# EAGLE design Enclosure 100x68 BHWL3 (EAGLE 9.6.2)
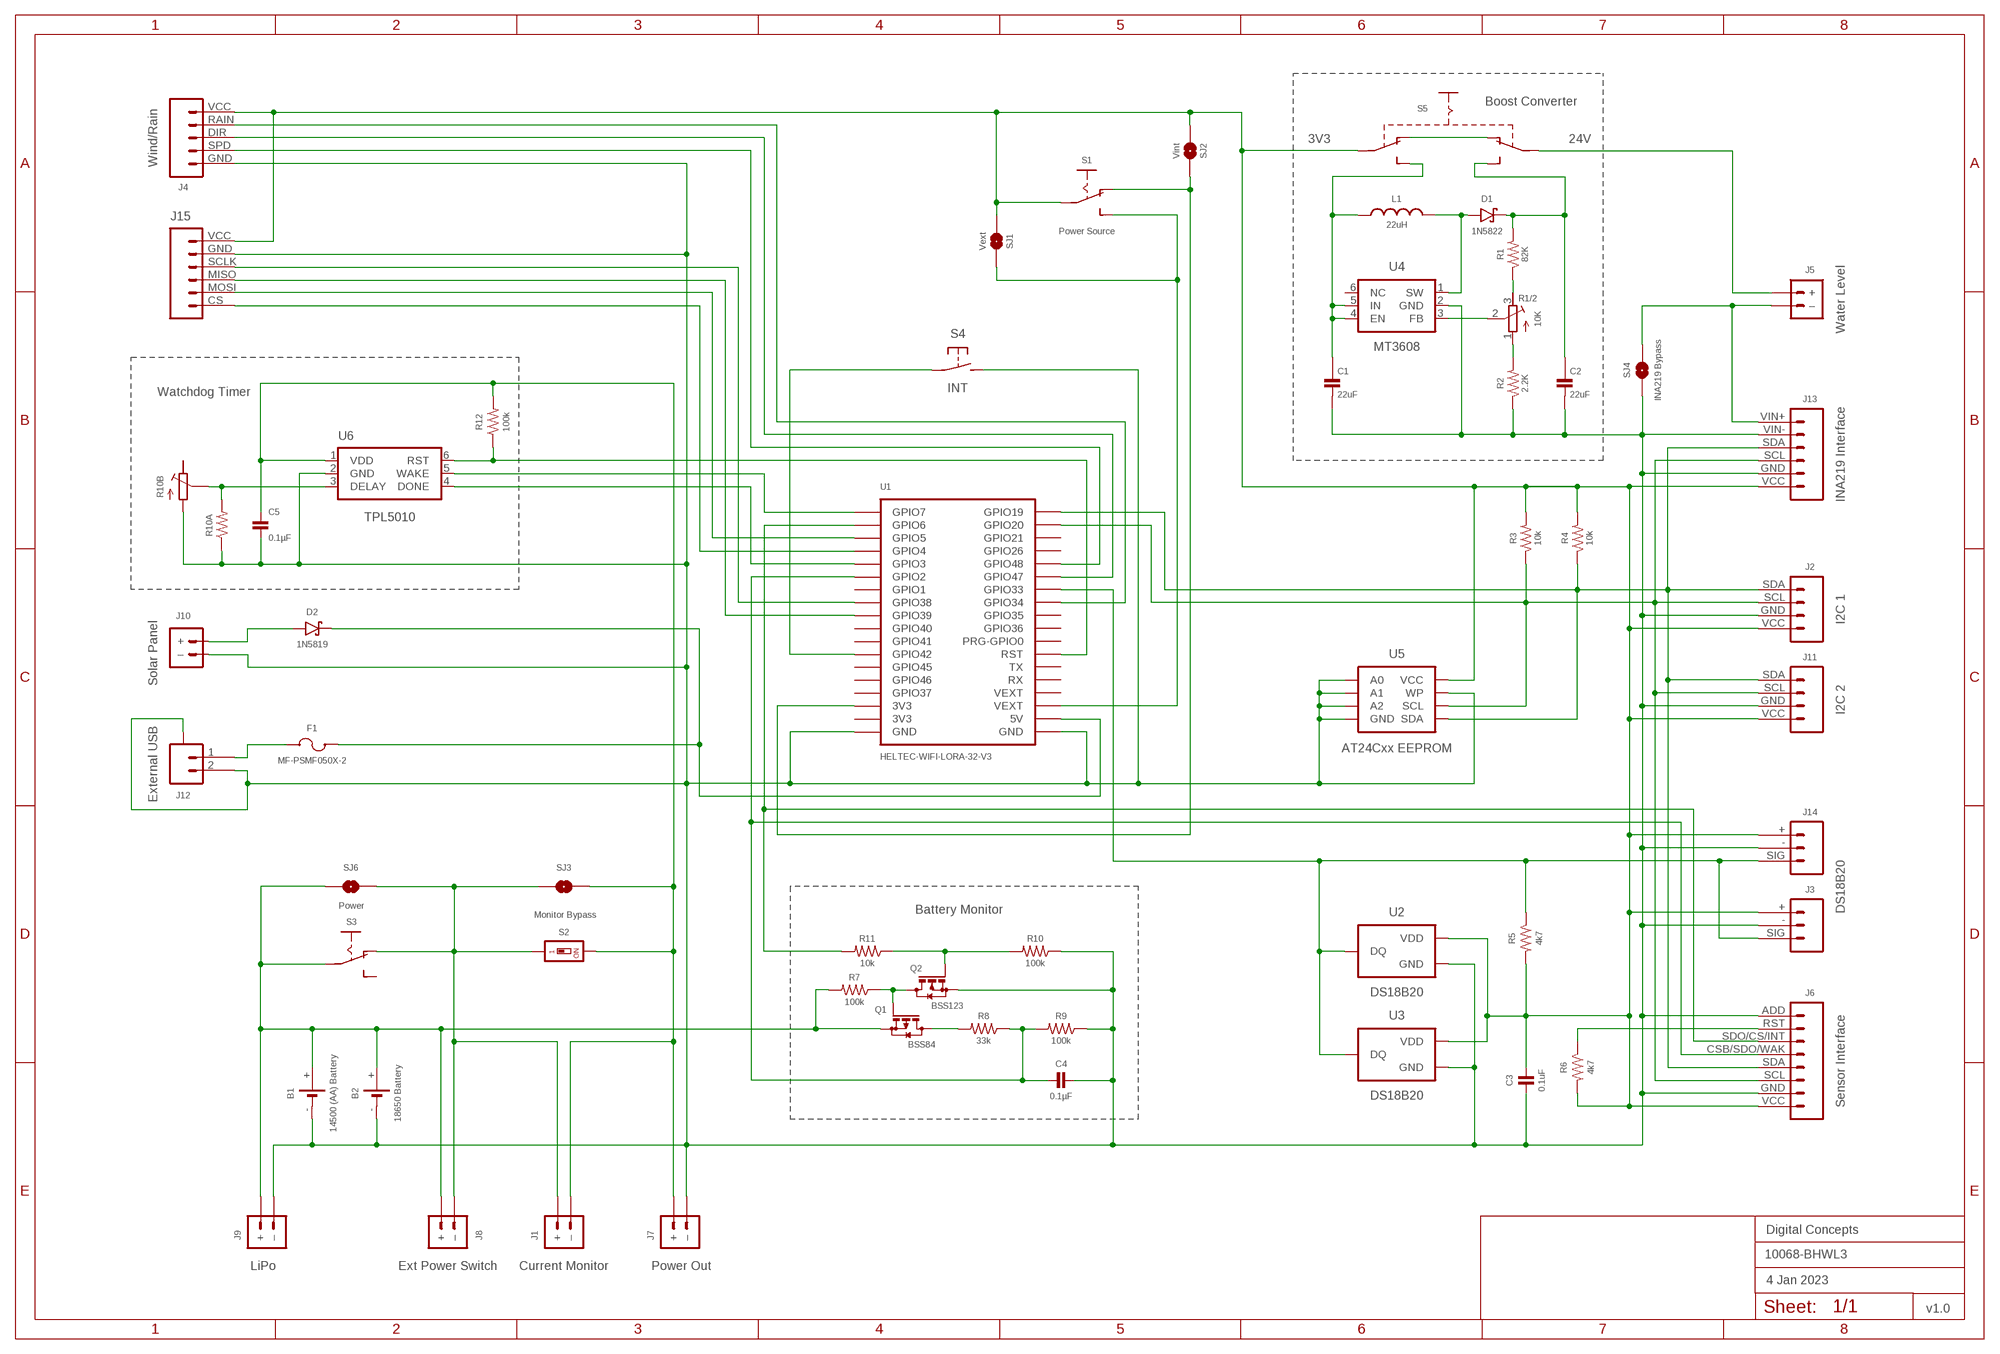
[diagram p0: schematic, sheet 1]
FRAME2 (A3L-LOC): DATE: 4 Jan 2023; OWNER: Digital Concepts; TITLE: 10068-BHWL3; VERSION: v1.0

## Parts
B1  14500 (AA) Battery  BATTERY-HOLDER-14500(AA)  [BATTERY-14500]
B2  18650 Battery  BATTERY-HOLDER-18650  [BATTERY-18650]
C1  22uF  CAPACITOR-1206  [C1206]
C2  22uF  CAPACITOR-1206  [C1206]
C3  0.1uF  CAPACITOR-0805  [C0805]
C4  0.1µF  CAPACITOR-0805  [C0805]
C5  0.1µF  CAPACITOR-0805  [C0805]
D1  1N5822  DIODE-SCHOTTKY-1N5822  [DIODE_SMB]
D2  1N5819  1N5819-SOD-123  [SOD-123]
F1  MF-PSMF050X-2  [F0805]
J1  Current Monitor  JST-PH2.0-2-HORIZONTALJST-PTH-2  [JST-PH2.0-2-HORIZONTAL]
J2  I2C 1  JST-PH2.0-4-VERTICAL-I2C  [JST-PH2.0-4-VERTICAL-I2C]
J3  DS18B20  JST-PH2.0-3-VERTICAL-DS18B20  [JST-PH2.0-3-VERTICAL-SIG]
J4  Wind/Rain  JST-PH2.0-5-DUAL-WEATHER  [JST-PH2.0-5-DUAL-WEATHER]
J5  Water Level  JST-PH2.0-2-DUAL-POWERJST-PTH-2  [JST-PH2.0-2-DUAL-POWER]
J6  Sensor Interface  HEADER-1X8-SENSOR  [CONN_08-SENSOR]
J7  Power Out  JST-GH1.25-2-HORIZONTAL-POWER  [JST-GH1.25-2-HORIZONTAL]
J8  Ext Power Switch  JST-PH2.0-2-DUAL-POWERJST-PTH-2  [JST-PH2.0-2-DUAL-POWER]
J9  LiPo  JST-PH2.0-2-HORIZONTAL-POWERJST-PTH-2  [JST-PH2.0-2-HORIZONTAL-POWER]
J10  Solar Panel  JST-PH2.0-2-VERTICAL  [JST-PH2.0-2-VERTICAL=POWER]
J11  I2C 2  JST-PH2.0-I2C-MALE-HORIZONTAL  [JST-PH2.0-4-HORIZONTAL]
J12  External USB  JST-SH1.0-2-SMD-HORIZONTAL  [JST-SH1.0-2-HORIZONTAL]
J13  INA219 Interface  INA219-I2C-MODULE  [CONN_06-INA219]
J14  JST-PH2.0-3-HORIZONTAL-DS18B20  [JST-PH2.0-DS18B20-HORIZONTAL]
J15  JST-PH2.0-6-HORIZONTAL-SPI  [JST-PH2.0-6-HORIZONTAL-SPI]
L1  22uH  INDUCTOR-CDRH104R/6D28L5038P  [CDRH104R+6D28]
Q1  BSS84  [SOT23-3]
Q2  BSS123  MOSFET-BSS123  [SOT23-3]
R1  82K  RESISTORR0805  [R0805]
R1/2  10K  RESISTOR-TRIMM-BAOTER-HORIZONTAL  [RTRIM64P]
R2  2.2K  RESISTORR0805  [R0805]
R3  10k  RESISTORR0805  [R0805]
R4  10k  RESISTORR0805  [R0805]
R5  4k7  RESISTORR0805  [R0805]
R6  4k7  RESISTORR0805  [R0805]
R7  100k  RESISTORR0805  [R0805]
R8  33k  RESISTORR0805  [R0805]
R9  100k  RESISTORR0805  [R0805]
R10  100k  RESISTORR0805  [R0805]
R10A  RESISTORR0805  [R0805]
R10B  RESISTOR-TRIMM-33  [RTRIM3*3]
R11  10k  RESISTORR0805  [R0805]
R12  100k  RESISTORR0805  [R0805]
S1  Power Source  SWITCH-SLIDE-SPDT-SMT  [SWITCH-SPDT-SMT]
S2  Monitor Bypass  SWITCH-DIP-SWS001  [SMD-001]
S3  Power  SWITCH-SLIDE-SPDT-PTH  [SWITCH-SPDT-PTH]
S4  INT  SWITCH-MOMENTARY-2-PIN  [SWITCH-2-PAD]
S5  SWITCH-SLIDE-DPDT-PTH-S  [SWITCH-DPDT-PTH]
SJ1  Vext  SJ  [SJ]
SJ2  Vint  SJ-V-2  [SJ-VIA-2]
SJ3  Monitor  SJ  [SJ]
SJ4  INA219 Bypass  SJ  [SJ]
SJ6  Power  SJ  [SJ]
U1  HELTEC-WIFI-LORA-32-V3  [HELTEC-WIFI-LORA-32-V3]
U2  DS18B20  THERMOMETER-DS18B20  [TO-92]
U3  DS18B20  THERMOMETER-DS18B20  [TO-92]
U4  MT3608  [SOT-23-6@1]
U5  AT24Cxx EEPROM  AT24CXX-EEPROM  [SOP-8]
U6  TPL5010  TPL5010DDCR  [SOT-23-6]

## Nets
GND: B1.- B2.- C1.2 C2.2 C3.2 C4.2 C5.2 J2.GND J3.- J4.GND J6.ADD J6.GND J7.-(–) J9.-(–) J10.-(–) J11.GND J12.2 J12.A@1(A) J12.A@2(A) J13.GND J13.VIN- J14.- J15.GND Q2.2(S) R2.1 R9.1 R10.1 R10A.1 R10B.1(A) S4.P$2(S) SJ4.1 U1.GND@1(GND) U1.GND@36(GND) U2.1(GND) U3.1(GND) U4.2(GND) U5.P$1(A0) U5.P$2(A1) U5.P$3(A2) U5.P$4(GND) U5.P$7(WP) U6.2(GND)
N$1: D2.A J10.+
N$2: J3.SIG J14.SIG R5.1 U1.GPIO33 U2.2(DQ) U3.2(DQ)
N$3: C4.1 J6.CSB/SDO/WAK R8.1 R9.2 U1.GPIO2
N$4: J2.SCL J6.SCL J11.SCL J13.SCL R3.1 U1.GPIO20 U5.P$6(SCL)
N$5: D2.C F1.1 U1.5V
N$6: D1.A L1.1 U4.1(SW)
N$7: Q1.3(D) R8.2
N$9: J6.RST R6.1
N$10: C5.1 J1.2(–) J7.+ R12.2 S2.2 SJ3.1 U6.1(VDD)
N$11: J2.SDA J6.SDA J11.SDA J13.SDA R4.1 U1.GPIO19 U5.P$5(SDA)
N$12: U1.GPIO7 U6.5(WAKE)
N$13: S1.3(S) SJ1.1 U1.VEXT@3(VEXT)
N$14: F1.2 J12.1
N$15: J5.-(–) J13.VIN+ SJ4.2
N$16: S4.P$1(P) U1.GPIO42
N$17: R1.1 R1/2.3(E)
N$18: R10A.2 R10B.2(S) U6.3(DELAY)
N$19: S1.1(O) SJ2.1 U1.3V3@34(3V3)
N$20: J5.+ S5.P$2(P1)
N$21: J1.1(+) J8.-(–) S2.1 S3.1(O) SJ3.2 SJ6.1
N$22: R1/2.2(S) U4.3(FB)
N$23: R1/2.1(A) R2.2
N$24: U1.GPIO3 U6.4(DONE)
N$25: C1.1 L1.2 S5.P$6(S2) U4.4(EN) U4.5(IN)
N$26: S5.P$1(O1) S5.P$4(O2)
N$27: J15.SCLK U1.GPIO38
N$28: C2.1 D1.C R1.2 S5.P$3(S1)
N$29: J15.MOSI U1.GPIO5
N$30: B1.+ B2.+ J8.+ J9.+ Q1.2(S) R7.2 S3.2(P) SJ6.2
N$31: J15.MISO U1.GPIO39
N$32: J6.SDO/CS/INT R11.2 U1.GPIO6
N$33: J15.CS U1.GPIO4
N$34: R12.1 U1.RST U6.6(RST)
N$35: Q1.1(G) Q2.3(D) R7.1
N$37: Q2.1(G) R10.2 R11.1
N$38: J4.SPD U1.GPIO48
N$39: J4.DIR U1.GPIO47
N$40: J4.RAIN U1.GPIO34
VEXT: C3.1 J2.VCC J3.+ J4.VCC J6.VCC J11.VCC J13.VCC J14.+ J15.VCC R3.2 R4.2 R5.2 R6.2 S1.2(P) S5.P$5(P2) SJ1.2 SJ2.2 SJ2.2@V U2.3(VDD) U3.3(VDD) U5.P$8(VCC)
Unconnected: R10B.3(E) S3.3(S) U1.3V3@35(3V3) U1.GPIO0(PRG-GPIO0) U1.GPIO1 U1.GPIO21 U1.GPIO26 U1.GPIO35 U1.GPIO36 U1.GPIO37 U1.GPIO40 U1.GPIO41 U1.GPIO45 U1.GPIO46 U1.RX U1.TX U1.VEXT@4(VEXT) U4.6(NC)

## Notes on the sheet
- Boost Converter
- 3V3 | 24V
- Watchdog Timer
- Battery Monitor

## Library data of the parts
B1 = digitalconcepts:BATTERY-HOLDER-14500(AA): 14500 (AA) battery holder
B2 = digitalconcepts:BATTERY-HOLDER-18650: 18650 Battery Holder
C1 C2 = digitalconcepts:CAPACITOR-1206: 1206 Capacitor
C3-C5 = digitalconcepts:CAPACITOR-0805: 0805 Capacitor
D1 = digitalconcepts:DIODE-SCHOTTKY-1N5822: 1N5822 Schottky Diode SMB
D2 = digitalconcepts:1N5819-SOD-123: 1N5819 Schottky Diode SOD-123
F1 = digitalconcepts:MF-PSMF050X-2: PTC Resettable Fuse
J1 = digitalconcepts:JST-PH2.0-2-HORIZONTAL: PH2.0 2P Right Angle PCB Connector; PROD_ID: CONN-09863; SKU: PRT-09914
J2 = digitalconcepts:JST-PH2.0-4-VERTICAL-I2C: PH2.0 4P I2C Vertical Connector
J3 = digitalconcepts:JST-PH2.0-3-VERTICAL-DS18B20: DS18B20 PH2.0 Vertical PCB Connector
J4 = digitalconcepts:JST-PH2.0-5-DUAL-WEATHER: PH2.0 5P Dual Connector
J5 J8 = digitalconcepts:JST-PH2.0-2-DUAL-POWER: JST PH2.0 2P PTH Dual-Side Connector (Power); PROD_ID: CONN-09863; SKU: PRT-09914
J6 = digitalconcepts:HEADER-1X8-SENSOR: IoT Sensors 1x8 Pin Header for 'Sandwich' IoT Sensors
J7 = digitalconcepts:JST-GH1.25-2-HORIZONTAL-POWER: JST GH1.25 2P PTH Connector (Power)
J9 = digitalconcepts:JST-PH2.0-2-HORIZONTAL-POWER: PH2.0 2P Right Angle PCB Connector; PROD_ID: CONN-09863; SKU: PRT-09914
J10 = digitalconcepts:JST-PH2.0-2-VERTICAL: PH2.0 2P PCB Connector
J11 = digitalconcepts:JST-PH2.0-I2C-MALE-HORIZONTAL: PH2.0 4P (I2C) Right Angle PCB Connector
J12 = digitalconcepts:JST-SH1.0-2-SMD-HORIZONTAL: JST SH1.0 2P SMD Horizontal Connector
J13 = digitalconcepts:INA219-I2C-MODULE: INA219 I2C Module
J14 = digitalconcepts:JST-PH2.0-3-HORIZONTAL-DS18B20: DS18B20 PH2.0 Right Angle PCB Connector
J15 = digitalconcepts:JST-PH2.0-6-HORIZONTAL-SPI: PH2.0 6P Horizontal Connector—SPI
L1 = digitalconcepts:INDUCTOR-CDRH104R/6D28: Inductor; SPICEPREFIX: L
Q1 = digitalconcepts:BSS84: P-CHANNEL MOS FET
Q2 = digitalconcepts:MOSFET-BSS123: N-CHANNEL MOS FET
R1-R10 R10A R11 R12 = digitalconcepts:RESISTOR: Resistor; SPICEPREFIX: R
R1/2 = digitalconcepts:RESISTOR-TRIMM-BAOTER-HORIZONTAL: Trimm Resistor - Horizontal BAOTER
R10B = digitalconcepts:RESISTOR-TRIMM-3*3: Trimm Resistor - 3*3 SMD
S1 = digitalconcepts:SWITCH-SLIDE-SPDT-SMT: Mini Sliding Switch SPDT SMT
S2 = digitalconcepts:SWITCH-DIP-SWS001: SMD Dip Switch 1 pol.
S3 = digitalconcepts:SWITCH-SLIDE-SPDT-PTH: Mini Sliding Switch SPDT PTH
S4 = digitalconcepts:SWITCH-MOMENTARY-2-PIN: 2 Pin Momentary Switch
S5 = digitalconcepts:SWITCH-SLIDE-DPDT-PTH-S: Switch DPDT PTH-S
SJ1 SJ3 SJ4 SJ6 = digitalconcepts:SJ: Solder Jumper
SJ2 = digitalconcepts:SJ-V-2: Solder Jumper with Pad Vias
U1 = digitalconcepts:HELTEC-WIFI-LORA-32-V3: Heltec WiFi LoRa 32 Development Board V3
U2 U3 = digitalconcepts:THERMOMETER-DS18B20: Digital Thermometer -55C-125C TO92-3; AVAILABILITY: Bad; DESCRIPTION: Temperature Sensor Digital, Local -55°C ~ 125°C 12 b 8-uMAX; MF: Maxim Integrated; MP: DS18B20; PACKAGE: TO-92 Maxim Integrated; PRICE: None
U4 = digitalconcepts:MT3608: MT3608 DC-DC Step-Up Voltage Converter
U5 = digitalconcepts:AT24CXX-EEPROM: AT24Cxx EEPROM SOP-8
U6 = digitalconcepts:TPL5010DDCR: TPL5010 Nano-Power System Timer with Watchdog

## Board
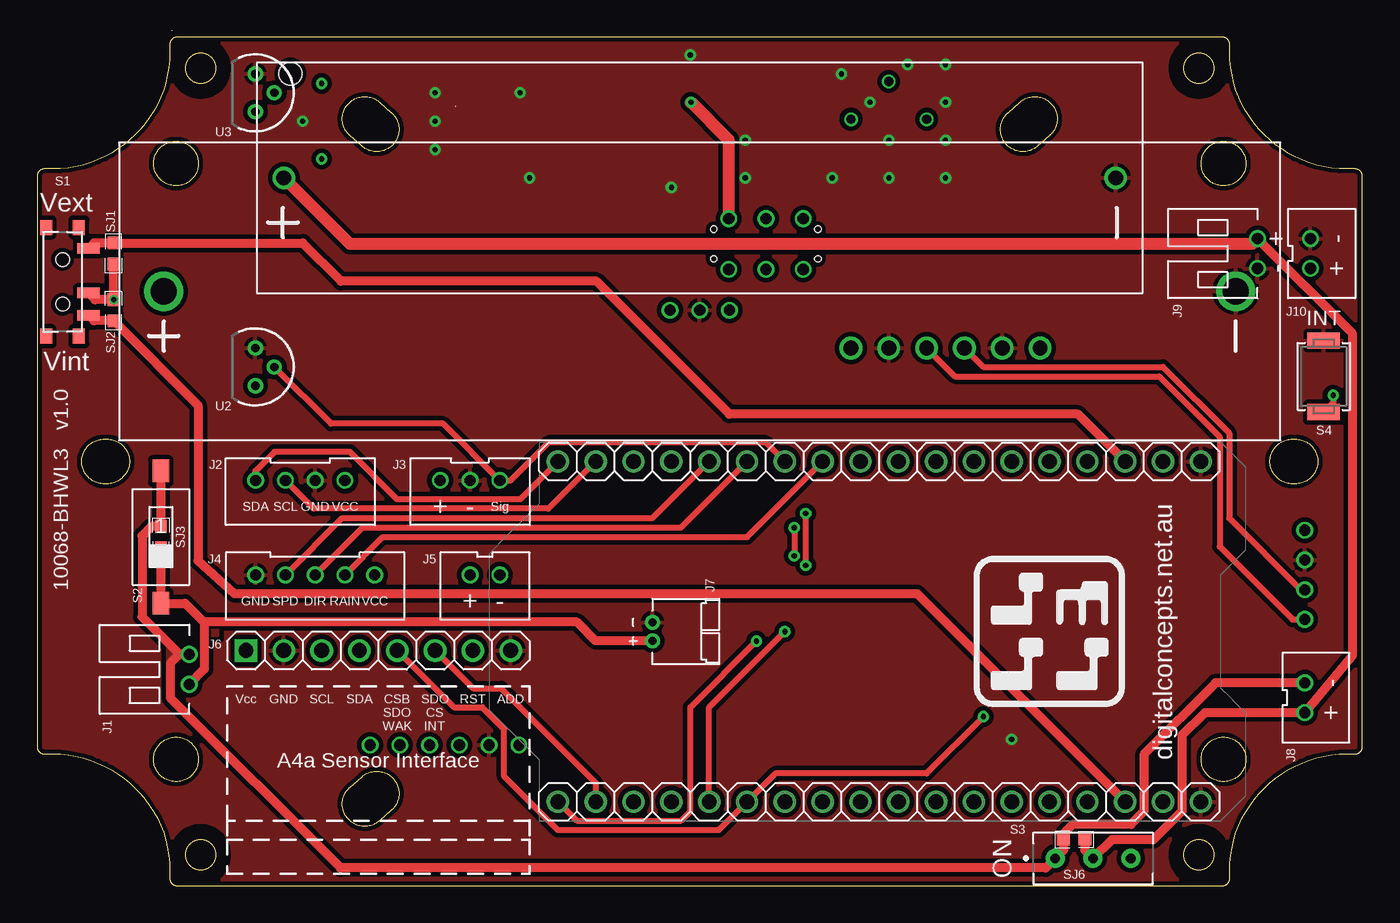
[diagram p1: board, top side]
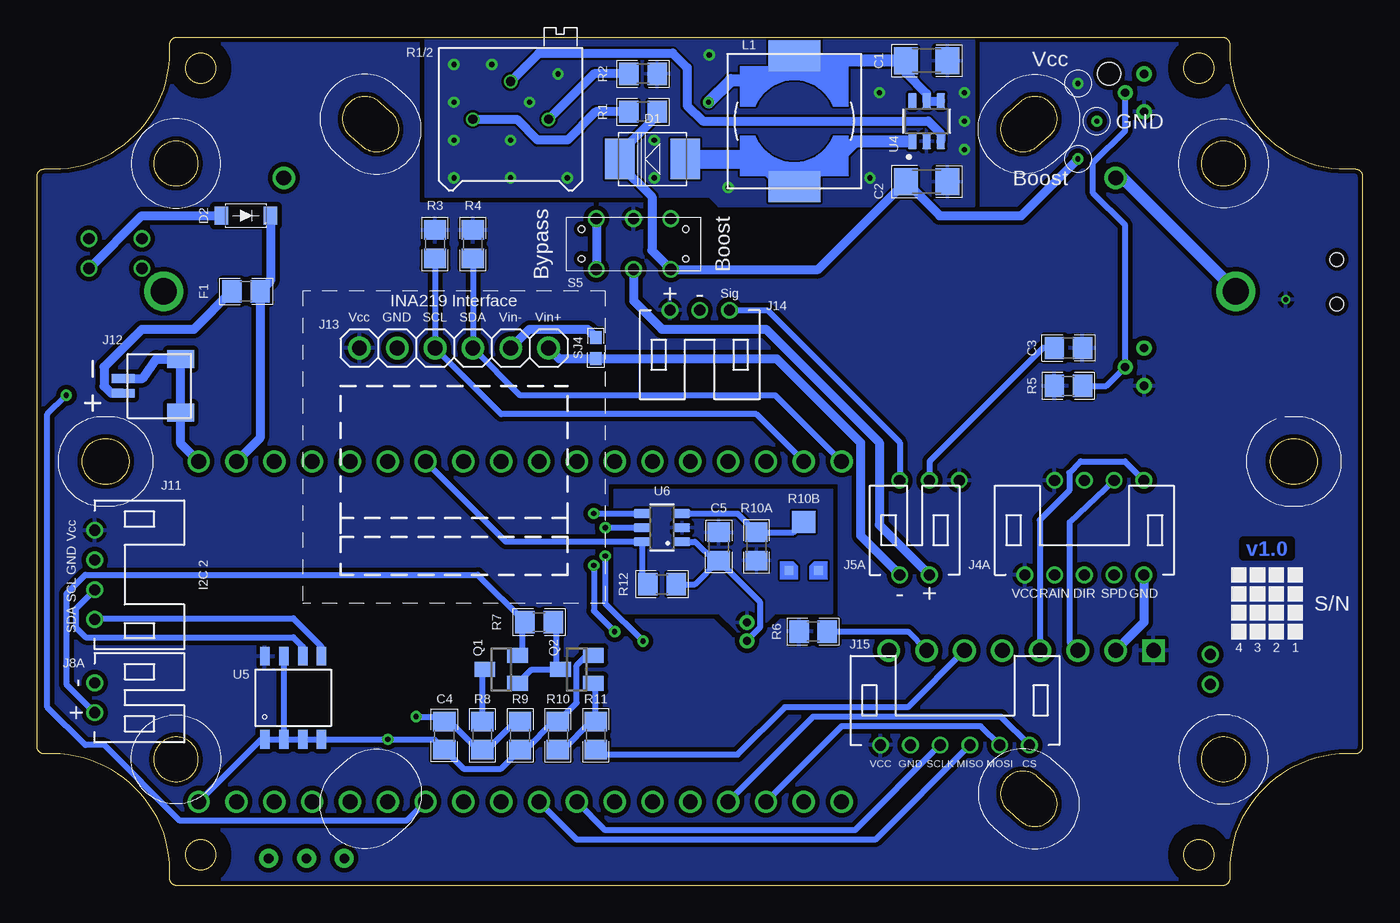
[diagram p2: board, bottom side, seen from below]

Size 89 x 57 mm. Coordinates in mm from the lower left corner, seen from the top.
Outline: 1134 segments
Outline: circle at 10.97,2.08 radius 1.02
Outline: circle at 10.97,54.92 radius 1.02
Outline: circle at 78.03,54.92 radius 1.02
Outline: circle at 78.03,2.08 radius 1.02
Copper layers (1*16): Top 0.035mm / dielectric 1.5mm / Bottom 0.035mm
Design rules "default *": minimum track width 6mil, minimum drill 0.35mm, track to track 6mil, track to pad 6mil, pad to pad 6mil, via to via 6mil, smd to smd 6mil, copper to edge 6mil, drill to drill 6mil, minimum pad ring 1mil, minimum via ring 8mil, stop-mask expansion 4mil, vias tented up to drill 0mil, thermal gap 10mil

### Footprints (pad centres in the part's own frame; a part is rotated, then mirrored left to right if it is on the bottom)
BATTERY-14500 = drill 1: + -27.94,0; - 27.94,0 | hole 1.524: -27.5,7
BATTERY-18650 = drill 1.75: + -36,0; - 36,0
C1206 = smd 1.6 x 1.8: 1 -1.4,0; 2 1.4,0
C0805 = smd 1.3 x 1.5: 1 -0.95,0; 2 0.95,0
DIODE_SMB = smd 2 x 2.7: A 2.2,0; C -2.2,0
SOD-123 = smd 0.91 x 1.22: A -1.65,0; C 1.65,0
F0805 = smd 1.3 x 1.5: 1 -0.95,0; 2 0.95,0
JST-PH2.0-2-HORIZONTAL = drill 0.75: 1 1,0; 2 -1,0
JST-PH2.0-4-VERTICAL-I2C = drill 0.75: GND 1,0; SCL -1,0; SDA -3,0; VCC 3,0
JST-PH2.0-3-VERTICAL-SIG = drill 0.75: + -2,0; - 0,0; SIG 2,0
JST-PH2.0-5-DUAL-WEATHER = drill 0.75: DIR 0,0; GND 4,0; RAIN -2,0; SPD 2,0; VCC -4,0
JST-PH2.0-2-DUAL-POWER = drill 0.75: + 1,0; - -1,0
CONN_08-SENSOR = drill 1 pad 1.524: ADD 17.78,0; CSB/SDO/WAK 10.16,0; GND 2.54,0; RST 15.24,0; SCL 5.08,0; SDA 7.62,0; SDO/CS/INT 12.7,0 | drill 1 pad 1.524 square: VCC 0,0
JST-GH1.25-2-HORIZONTAL = drill 0.55 pad 1.016: + -0.625,0; - 0.625,0
JST-PH2.0-2-HORIZONTAL-POWER = drill 0.75: + 1,0; - -1,0
JST-PH2.0-2-VERTICAL=POWER = drill 0.75: + -1,0; - 1,0
JST-PH2.0-4-HORIZONTAL = drill 0.75: GND -1,0; SCL 1,0; SDA 3,0; VCC -3,0
JST-SH1.0-2-HORIZONTAL = smd 0.6 x 1.55: 1 -0.5,2.54; 2 0.5,2.54 | smd 1.2 x 1.8: A@1 -1.8,-1.335; A@2 1.8,-1.335
CONN_06-INA219 = drill 1 pad 1.524: GND 2.54,0; SCL 5.08,0; SDA 7.62,0; VCC 0,0; VIN+ 12.7,0; VIN- 10.16,0
JST-PH2.0-DS18B20-HORIZONTAL = drill 0.75: + 2,0; - 0,0; SIG -2,0
JST-PH2.0-6-HORIZONTAL-SPI = drill 0.75: CS 5,0; GND -3,0; MISO 1,0; MOSI 3,0; SCLK -1,0; VCC -5,0
CDRH104R+6D28 = smd 2.1 x 3.5: 1 -4.4,0; 2 4.4,0
SOT23-3 = smd 1 x 1.4: 1 -0.95,-1.1; 2 0.95,-1.1; 3 0,1.1
R0805 = smd 1.3 x 1.5: 1 -0.95,0; 2 0.95,0
RTRIM64P = drill 0.61: 1 0,-2.54; 2 2.54,0; 3 0,2.54
RTRIM3*3 = smd 0.6 x 0.6: 1 -1,-1.6; 3 1,-1.6 | smd 1.6 x 1.5: 2 0,1.65
SWITCH-SPDT-SMT = smd 0.7 x 1.5: 1 2.25,1.75; 2 0.75,1.75; 3 -2.25,1.75 | smd 1 x 0.8: GND@1 3.65,-1.1; GND@2 3.65,1.1; GND@3 -3.65,1.1; GND@4 -3.65,-1.1 | hole 0.9: -1.5,0; 1.5,0
SMD-001 = smd 1.1 x 1.5: 1 0,-4.45; 2 0,4.45
SWITCH-SPDT-PTH = drill 0.65 pad 1.27: 1 -2.54,0; 2 0,0; 3 2.54,0
SWITCH-2-PAD = smd 1.067 x 2.184: P$1 -2.4,0; P$2 2.4,0
SWITCH-DPDT-PTH = drill 0.75: P$1 -1.7,2.5; P$2 -1.7,0; P$3 -1.7,-2.5; P$4 1.7,2.5; P$5 1.7,0; P$6 1.7,-2.5 | hole 0.42: 1,3.5; -1,3.5; 1,-3.5; -1,-3.5
SJ = smd 0.864 x 0.762: 1 -0.711,0; 2 0.711,0
SJ-VIA-2 = smd 0.864 x 0.762: 1 -0.711,0; 2 0.711,0 | drill 0.35 pad 0.61: 2@V 0.711,0
HELTEC-WIFI-LORA-32-V3 = drill 1: 3V3@34 -22.86,5.08; 3V3@35 -22.86,2.54; 5V 0,2.54; GND@1 0,0; GND@36 -22.86,0; GPIO0 0,17.78; GPIO1 -22.86,27.94; GPIO2 -22.86,30.48; GPIO3 -22.86,33.02; GPIO4 -22.86,35.56; GPIO5 -22.86,38.1; GPIO6 -22.86,40.64; GPIO7 -22.86,43.18; GPIO19 0,43.18; GPIO20 0,40.64; GPIO21 0,38.1; GPIO26 0,35.56; GPIO33 0,27.94; GPIO34 0,25.4; GPIO35 0,22.86; GPIO36 0,20.32; GPIO37 -22.86,7.62; GPIO38 -22.86,25.4; GPIO39 -22.86,22.86; GPIO40 -22.86,20.32; GPIO41 -22.86,17.78; GPIO42 -22.86,15.24; GPIO45 -22.86,12.7; GPIO46 -22.86,10.16; GPIO47 0,30.48; GPIO48 0,33.02; RST 0,15.24; RX 0,10.16; TX 0,12.7; VEXT@3 0,5.08; VEXT@4 0,7.62
TO-92 = drill 0.55 pad 1.016: 1 -1.27,0; 2 0,1.27; 3 1.27,0
SOT-23-6@1 = smd 1.1 x 0.6: 1 -1.35,0.95; 2 -1.35,0; 3 -1.35,-0.95; 4 1.35,-0.95; 5 1.35,0; 6 1.35,0.95
SOP-8 = smd 0.635 x 1.27: P$1 -1.905,-2.794; P$2 -0.635,-2.794; P$3 0.635,-2.794; P$4 1.905,-2.794; P$5 1.905,2.794; P$6 0.635,2.794; P$7 -0.635,2.794; P$8 -1.905,2.794
SOT-23-6 = smd 1.1 x 0.6: 1 -1.35,0.95; 2 -1.35,0; 3 -1.35,-0.95; 4 1.35,-0.95; 5 1.35,0; 6 1.35,0.95

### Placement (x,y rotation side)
B1  44.5,47.55 0 top
B2  44.5,39.93 0 top
C1  29.26,55.42 0 bottom
C2  29.26,47.3 0 bottom
C3  19.73,36.12 180 bottom
C4  61.64,10.08 270 bottom
C5  43.23,22.78 90 bottom
D1  47.67,48.82 0 bottom
D2  74.98,45.01 0 bottom
F1  74.98,39.93 180 bottom
J1  10.21,14.53 90 top
J2  17.67,27.23 0 top
J3  29.07,27.23 0 top
J4  18.67,20.88 0 bottom
J5  30.07,20.88 0 bottom
J6  14.02,15.8 0 top
J7  41.32,17.07 90 top
J8  85.14,12.62 270 bottom
J9  81.96,42.47 90 top
J10  85.52,42.47 90 top
J11  85.14,20.88 270 bottom
J12  80.69,33.58 90 bottom
J13  67.36,36.12 0 bottom
J14  44.5,38.66 180 bottom
J15  27.35,9.45 0 bottom
L1  38.15,51.36 90 bottom
Q1  57.83,14.53 90 bottom
Q2  52.75,14.53 90 bottom
R1  48.31,51.99 0 bottom
R1/2  57.2,51.49 90 bottom
R2  48.31,54.53 180 bottom
R3  62.28,43.1 90 bottom
R4  59.74,43.1 90 bottom
R5  19.73,33.58 180 bottom
R6  36.88,17.07 180 bottom
R7  55.29,17.7 180 bottom
R8  59.1,10.08 90 bottom
R9  56.56,10.08 90 bottom
R10  54.02,10.08 270 bottom
R10A  40.69,22.78 90 bottom
R10B  37.51,22.78 0 bottom
R11  51.48,10.08 270 bottom
R12  47.04,20.24 0 bottom
S1  1.7,40.56 270 top
S2  8.3,23.42 180 top
S3  70.92,1.83 0 top
S4  86.41,34.21 90 top
S5  48.94,43.1 90 bottom
SJ1  5.13,42.47 270 top
SJ2  5.13,38.66 90 top
SJ3  8.3,23.42 90 top
SJ4  51.48,36.12 270 bottom
SJ6  69.65,3.1 0 top
U1  78.15,28.5 90 top
U2  14.65,34.85 270 top
U3  14.65,53.26 270 top
U4  29.26,51.36 90 bottom
U5  71.8,12.62 0 bottom
U6  47.04,24.05 180 bottom

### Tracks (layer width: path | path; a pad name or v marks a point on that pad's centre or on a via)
$X
  cutout Bottom: 10.97,56.95 arc180 10.97,52.88 arc180
$X1
  cutout Bottom: 78.03,56.95 arc180 78.03,52.88 arc180
$X2
  cutout Top: 78.03,4.12 arc180 78.03,0.05 arc180
$X3
  cutout Top: 10.97,4.12 arc180 10.97,0.05 arc180
$X4
  cutout Top: 10.97,56.95 arc180 10.97,52.88 arc180
$X5
  cutout Top: 78.03,56.95 arc180 78.03,52.88 arc180
$X6
  cutout Bottom: 78.03,4.12 arc180 78.03,0.05 arc180
$X7
  cutout Bottom: 10.97,4.12 arc180 10.97,0.05 arc180
GND  (via drill 0.35)
  Bottom 0.406: U5.P$7 U5.P$2 | U5.P$2 U5.P$1 73.96,9.83 U1.GND@36 | U5.P$2 U5.P$3 U5.P$4 v65.45,9.83 62.34,9.83 C4.2 60.37,7.86 57.83,7.86 R9.1 56.21,9.13 54.31,11.03 R10.1 52.76,12.3 52.76,14.81 52.09,15.48 Q2.2 | C3.2 21.45,36.12 29.07,28.5 J3.-
  Bottom 0.61: J12.2 81.93,34.08 81,35.38 J12.A@2 J12.A@1 79.36,29.7 U1.GND@1 | J4.GND 14.67,17.69 J6.GND | J13.VIN- 55.93,37.39 52.04,37.39 SJ4.1
  other vias: 26.72,53.26 54.02,54.53 55.93,52.63 47.55,50.09 47.55,47.55 53.39,47.55 57.2,47.55 57.2,50.09 61.01,47.55 61.01,50.09 61.01,55.17 26.72,51.36 58.47,55.17 61.01,52.63 43.86,55.8 32.43,53.26 33.07,47.55 26.72,49.45 17.83,51.36 42.59,46.91
  pour Top (isolate 0.305, rank 2): -1.65,58.87 -1.65,-1.92 90.59,-1.92 90.59,58.87
  pour Bottom: 26.08,57.07 26.08,45.64 43.23,45.64 43.86,46.28 62.91,46.28 62.91,57.07
  pour Bottom: 50.21,26.59 50.21,18.34 43.23,18.34 41.96,17.07 40.69,17.07 39.42,18.34 35.61,18.34 35.61,26.59
N$1
  Bottom 0.61: J10.+ 81.98,45.01 D2.A
N$2
  Top 0.406: U2.2 19.73,31.04 27.26,31.04 J3.SIG 31.8,27.23 34.34,29.77 48.94,29.77 U1.GPIO33
  Bottom 0.406: J3.SIG 31.07,29.77 39.96,38.66 J14.SIG | U3.2 15.92,50.72 18.08,48.57 18.08,46.53 15.92,44.37 U2.2 17.19,33.58 R5.1
N$3  (via drill 0.35)
  Top 0.406: J6.CSB/SDO/WAK 27.99,11.99 29.89,11.99 31.37,10.52 31.37,7.34 34.97,3.73 45.77,3.73 U1.GPIO2 49.58,7.54 59.74,7.54 v63.55,11.35
  Bottom 0.406: R9.2 56.87,11.03 58.77,9.13 R8.1 59.38,9.13 61.29,11.03 C4.1 61.96,11.35 v63.55,11.35
N$4
  Top 0.406: J13.SCL 63.55,34.85 75.61,34.85 80.06,30.4 80.06,24.69 84.87,19.88 J11.SCL | J2.SCL 18.57,25.32 34.34,25.32 U1.GPIO20
  Bottom 0.406: J2.SCL 19.66,24.41 19.66,16.36 J6.SCL | U5.P$6 71.17,16.05 71.8,16.69 85.76,16.69 86.41,17.34 86.41,18.61 J11.SCL | R3.1 J13.SCL 57.83,31.67 40.69,31.67 U1.GPIO20
N$5
  Bottom 0.61: D2.C 73.33,40.63 F1.1 74.03,30.08 U1.5V
N$6
  Bottom 0.152: U4.1 30.4,50.01
  Bottom 0.813: 40.68,48.82 38.96,47.11 L1.1 36.84,48.27 35.79,48.27 34.05,50.01 30.4,50.01
  Bottom 1.27: D1.A 40.68,48.82
N$7
  Bottom 0.406: Q1.3 59.1,14.36 R8.2
N$8
  pour Top: 11.48,17.7 12.75,17.7 11.48,16.43
N$9
  Bottom 0.406: J6.RST 30.53,17.07 R6.1
N$10
  Top 0.61: J1.2 11.23,14.55 11.23,17.67 11.19,17.7 | J7.+ 37.51,16.44 36.25,17.7 11.19,17.7 | SJ3.1 S2.2 9.93,18.97 11.19,17.7
  Bottom 0.406: R12.2 44.82,20.24 C5.1 | U6.1 44.82,23.1 43.55,21.83 C5.1 | C5.1 40.46,19.07 40.46,17.34 41.32,16.47 J7.+
N$11
  Top 0.406: J13.SDA 61.64,34.21 75.36,34.21 79.42,30.15 79.42,22.78 84.33,17.88 J11.SDA | J2.SDA 14.67,27.86 15.94,29.13 21,29.13 24.18,25.96 32.43,25.96 U1.GPIO19
  Bottom 0.406: J6.SDA 21.66,15.82 21.66,24.56 19.68,26.54 19.68,27.73 18.92,28.5 15.94,28.5 J2.SDA | J11.SDA 85.06,17.96 71.8,17.96 69.9,16.05 U5.P$5 | R4.1 J13.SDA 56.56,32.94 39.42,32.94 U1.GPIO19
N$12  (via drill 0.35)
  Top 0.406: v48.31,16.43 43.86,11.99 43.86,5 43.23,4.37 36.24,4.37 U1.GPIO7 | v50.85,24.05 v50.85,22.15
  Bottom 0.406: v50.85,24.05 U6.5 | v50.85,22.15 50.85,18.97 v48.31,16.43
N$13
  Top 0.61: S1.3 3.82,43.18 SJ1.1 17.83,43.18 20.41,40.6 37.55,40.6 46.48,31.67 69.9,31.67 U1.VEXT@3
N$14
  Bottom 0.61: J12.1 84.02,33.08 84.5,33.56 84.5,34.85 81.96,37.39 78.47,37.39 F1.2
N$15
  Bottom 0.61: J5.- 33.7,23.51 33.7,29.77 39.34,35.41 SJ4.2 53.95,35.41 J13.VIN+
N$16  (via drill 0.35)
  Top 0.406: S4.P$1 87.04,32.45 v87.04,32.94
  Bottom 0.406: U1.GPIO42 64.18,4.37 79.42,4.37 84.5,9.45 85.77,9.45 88.31,11.99 88.31,31.67 v87.04,32.94
N$17
  Bottom 0.61: R1.1 51.48,51.99 53.39,50.09 55.38,50.09 56.78,51.49 R1/2.3
N$18
  Bottom 0.406: U6.3 41.96,25 R10A.2 38.21,23.73 R10B.2
N$19
  Top 0.61: S1.1 3.82,37.95 SJ2.1 10.81,32.27 10.81,21.82 13.24,19.61 59.1,19.61 U1.3V3@34
N$20
  Bottom 0.61: S5.P$2 48.94,39.29 47.04,37.39 40.05,37.39 32.43,29.77 32.43,24.24 J5.+
N$21
  Top 0.61: S2.1 SJ3.2 7.67,24.13 7.03,23.5 7.03,18.07 9.57,15.53 J1.1 9.55,15.53 8.94,14.92 8.94,12.62 20.37,1.19 67.74,1.19 S3.1 68.93,2.39 SJ6.1 68.93,3.48 69.57,4.12 73.46,4.12 74.34,5 74.34,8.81 79.15,13.62 J8.-
  pour Top (no thermals): 9.55,15.55 8.94,16.16 8.94,14.94
N$22
  Bottom 0.61: U4.3 28.31,50.51 29.16,51.36 44.3,51.36 45.35,52.41 45.35,54.95 46.33,55.93 55.29,55.93 R1/2.2
N$23
  Bottom 0.61: R2.2 51.61,54.53 R1/2.1
N$24  (via drill 0.35)
  Top 0.406: U1.GPIO3 45.13,11.99 v50.21,17.07 | v51.61,25 v51.61,21.51
  Bottom 0.406: v51.61,25 U6.4 | v51.61,21.51 51.61,18.47 v50.21,17.07
N$25  (via drill 0.35)
  Top 0.813: v43.9,52.63 46.44,50.09 S5.P$6
  Bottom 0.61: C1.1 30.66,54.61 29.26,53.21 U4.5 U4.4
  Bottom 0.813: C1.1 38.04,55.42 L1.2 38.99,55.36 39.98,54.12 42.41,54.12 v43.9,52.63
N$26
  Bottom 0.61: S5.P$4 S5.P$1
N$27
  Bottom 0.406: J15.SCLK 34.07,3.73 50.85,3.73 U1.GPIO38
N$28  (via drill 0.35)
  Bottom 0.61: v19.1,48.82 22.91,45.01 28.37,45.01 C2.1 36.55,41.4 S5.P$3 47.71,42.67 47.71,46.28 49.87,48.44 D1.C 49.87,49.23 47.36,51.74 R1.2
N$29
  Bottom 0.406: J15.MOSI 25.62,10.72 34.97,10.72 U1.GPIO5
N$30
  Top 0.61: SJ6.2 70.36,2.39 S3.2 72.19,3.1 74.98,3.1 76.88,5 76.88,10.08 78.42,11.62 J8.+ 88.31,15.43 88.31,37.12 J9.+
  Top 0.813: J9.+ 81.6,43.1 21,43.1 B1.+
  Bottom 0.406: Q1.2 56.44,15.78 56.44,17.51 R7.2 59.42,20.88 85.77,20.88 87.04,19.61 87.04,13.53 J8.+
  Bottom 0.813: B1.+ 16.12,47.55 B2.+
N$31
  Bottom 0.406: J15.MISO 32.7,3.1 52.75,3.1 U1.GPIO39
N$32
  Top 0.406: U1.GPIO6 37.51,6.91 31.16,13.26 29.26,13.26 J6.SDO/CS/INT
  Bottom 0.406: R11.2 51.16,8.81 41.96,8.81 38.78,11.99 30.53,11.99 J6.SDO/CS/INT
N$33
  Bottom 0.406: J15.CS 24.26,11.35 36.88,11.35 U1.GPIO4
N$34
  Bottom 0.406: R12.1 48.39,20.64 U6.6 57.52,23.1 U1.RST
N$35
  Bottom 0.406: Q1.1 55.78,14.53 Q2.3 54.15,14.83 54.15,17.51 R7.1
N$37
  Bottom 0.406: R10.2 53.69,9.13 51.79,11.03 R11.1 51.48,13.41 Q2.1
N$38
  Top 0.406: J4.SPD 20.48,24.69 41.32,24.69 U1.GPIO48
N$39
  Top 0.406: J4.DIR 21.84,24.05 43.23,24.05 U1.GPIO47
N$40
  Top 0.406: J4.RAIN 23.21,23.42 47.67,23.42 U1.GPIO34
VEXT  (via drill 0.35)
  Top 0.61: S1.2 3.89,39.37 SJ2.2@V SJ1.2
  other vias: 19.1,53.9
  pour Bottom (isolate 0.305, rank 2): -0.65,57.87 -0.65,-0.92 89.59,-0.92 89.59,57.87

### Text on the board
Bottom: v1.0
tPlace: 10068-BHWL3 v1.0 | digitalconcepts.net.au | Vcc | GND | SCL | SDA | RST | ADD | CSB / SDO / WAK | SDO / CS / INT
bPlace: Vin+ | Vin- | SDA | SCL | GND | Vcc | S/N | 1 | 2 | 3 | 4
tNames: Vext | Vint | A4a Sensor Interface | ON
bNames: Vcc | GND | Boost | Boost | Bypass | Vcc | GND | J4A | J5A | SCL | SDA | J8A
bValues: Wind/Rain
